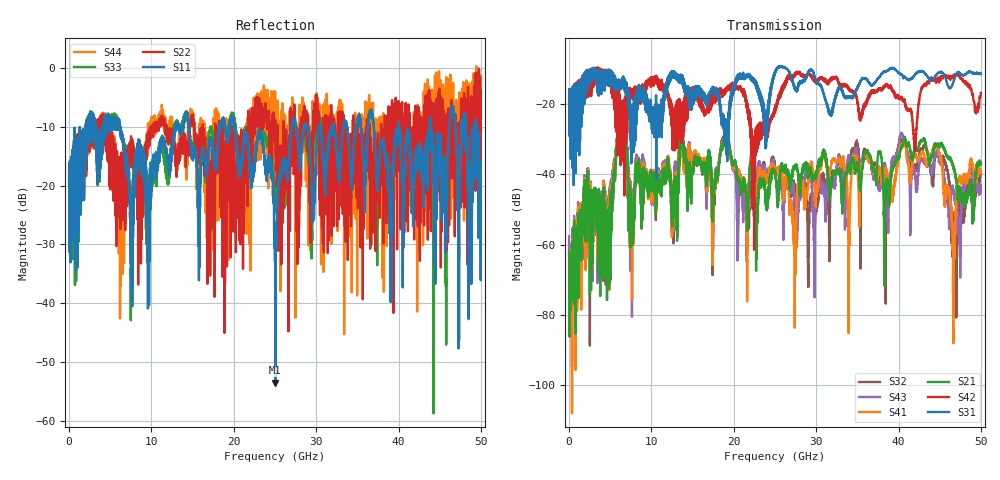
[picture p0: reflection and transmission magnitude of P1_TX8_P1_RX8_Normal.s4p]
!Keysight Technologies,N5225B,MY57041031,A.13.20.10
!Date: Friday, May 31, 2019 11:26:22
!Correction: S11(Full 4 Port(1,2,3,4))
!S12(Full 4 Port(1,2,3,4))
!S13(Full 4 Port(1,2,3,4))
!S14(Full 4 Port(1,2,3,4))
!S21(Full 4 Port(1,2,3,4))
!S22(Full 4 Port(1,2,3,4))
!S23(Full 4 Port(1,2,3,4))
!S24(Full 4 Port(1,2,3,4))
!S31(Full 4 Port(1,2,3,4))
!S32(Full 4 Port(1,2,3,4))
!S33(Full 4 Port(1,2,3,4))
!S34(Full 4 Port(1,2,3,4))
!S41(Full 4 Port(1,2,3,4))
!S42(Full 4 Port(1,2,3,4))
!S43(Full 4 Port(1,2,3,4))
!S44(Full 4 Port(1,2,3,4))
!S4P File: Measurements: <S11,S12,S13,S14>,
!<S21,S22,S23,S24>,
!<S31,S32,S33,S34>,
!<S41,S42,S43,S44>:
# Hz S  dB  R 50.0
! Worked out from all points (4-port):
!   5000 points, 10 MHz to 50 GHz, reference 50 ohm
!   strongest paths, dB at 10 MHz, 12.51 GHz, 25.01 GHz, 37.51 GHz, 50 GHz:
!     S31: -19.7, -10.8, -11.0, -12.6, -11.2
!     S42: -19.4, -24.3, -22.4, -16.1, -16.8
!     S21: -61.9, -50.5, -39.5, -34.6, -37.2
!     S41: -62.5, -49.5, -39.2, -39.2, -39.1
!     S43: -57.6, -51.1, -40.1, -43.3, -43.0
!     S32: -61.2, -53.5, -38.1, -41.4, -39.6
!   lowest |S11| = -53.4 dB at 25.05 GHz (marker M1), VSWR 1.00, Z = 49.8 - j0.0894 ohm
!   |S11| at or under -10 dB: 6.192 GHz to 12.89 GHz (6.695 GHz wide, 70.2 % of centre); 20.1 GHz to 26.99 GHz (6.891 GHz wide, 29.3 % of centre); 40 GHz to 43.76 GHz (3.761 GHz wide, 8.98 % of centre)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
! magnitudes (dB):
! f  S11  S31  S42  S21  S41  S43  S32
! 10 MHz  -19.4  -19.7  -19.4  -61.9  -62.5  -57.6  -61.2
! 6.19 GHz  -9.8  -13.7  -31.7  -26.3  -25.9  -25.5  -25.7
! 7.7 GHz  -25.4  -24.8  -16.9  -50.9  -60.4  -51.5  -47.6
! 25.05 GHz  -53.4  -10.5  -21.6  -41.0  -39.0  -40.0  -39.2
! 44.57 GHz  -20.0  -11.7  -13.9  -31.4  -32.3  -34.5  -34.3
! 46.69 GHz  -8.2  -13.4  -11.8  -37.6  -67.6  -44.4  -54.5
! 50 GHz  -22.7  -11.2  -16.8  -37.2  -39.1  -43.0  -39.6
